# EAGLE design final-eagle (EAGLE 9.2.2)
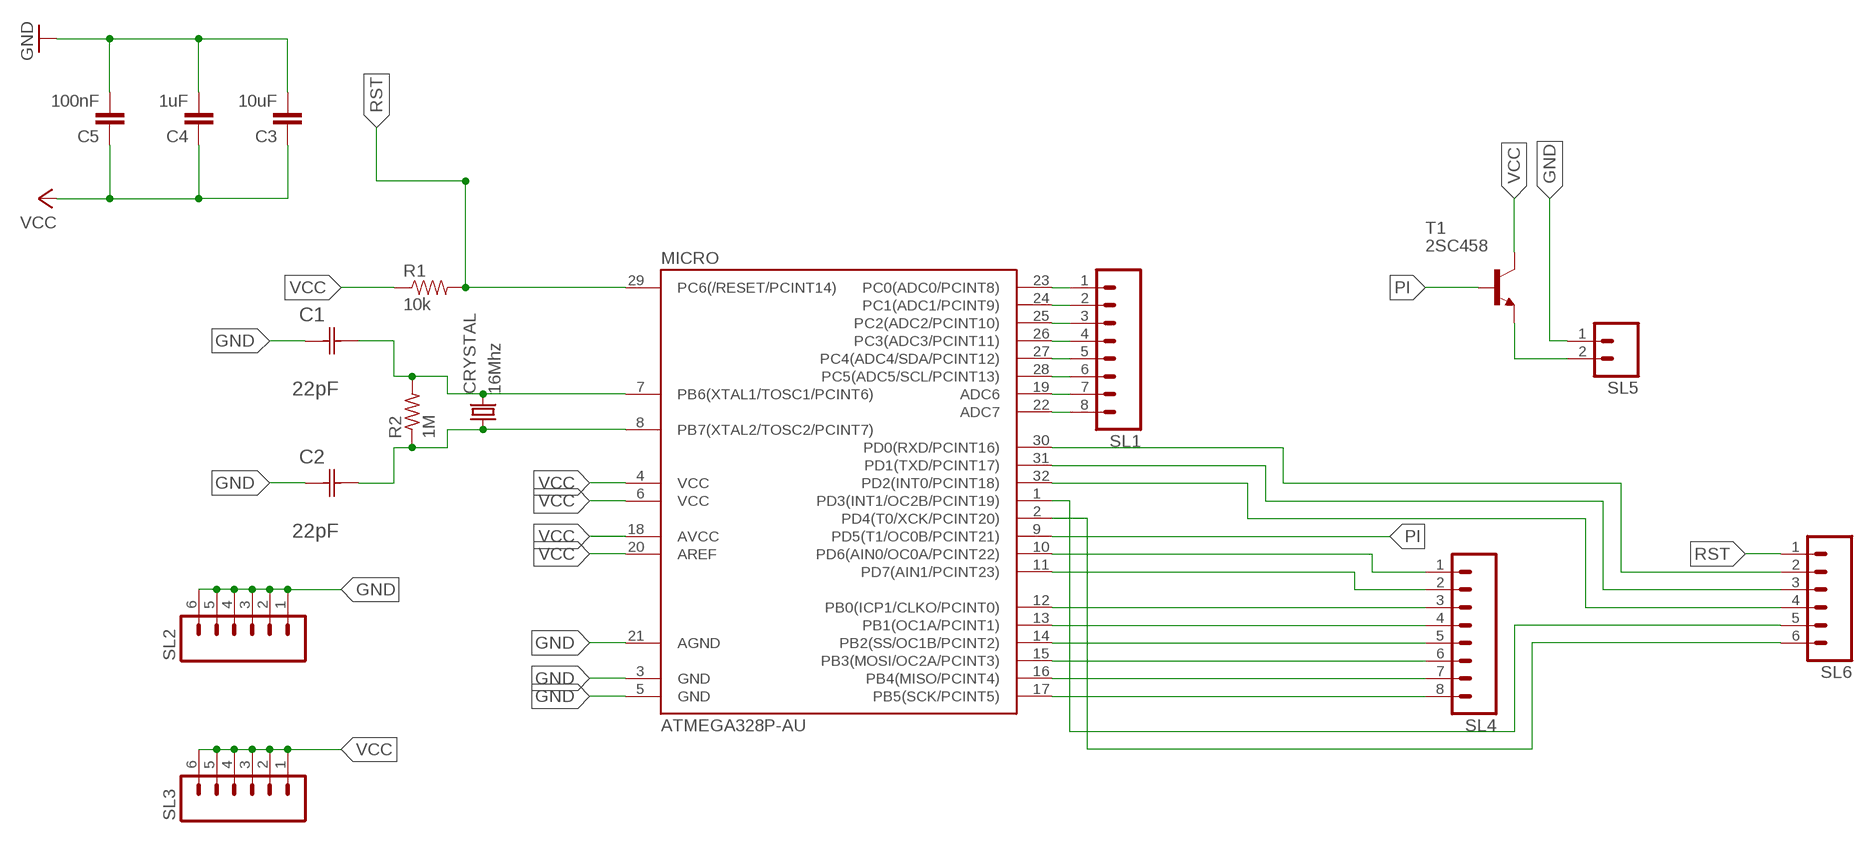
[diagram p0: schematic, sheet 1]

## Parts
C1  22pF  0612ZC225MAT2A  [CAPC3216X178N]
C2  22pF  0612ZC225MAT2A  [CAPC3216X178N]
C3  10uF  CAP1206  [1206]
C4  1uF  CAP1206  [1206]
C5  100nF  CAP1206  [1206]
CRYSTAL  16Mhz  CSM-7X-DU  [CSM-7X-DU]
MICRO  ATMEGA328P-AU  ATMEGA48/88/168-AU  [TQFP32-08]
R1  10k  RESISTOR1206  [1206]
R2  1M  RES-US1206FAB  [R1206FAB]
SL1  M08  [08P]
SL2  M06  [06P]
SL3  M06  [06P]
SL4  M08  [08P]
SL5  M02  [02P]
SL6  M06  [06P]
T1  2SC458  [TO92-ECB]

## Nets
GND: C1.1(C1) C2.1(C1) C3.2 C4.2 C5.2 MICRO.3(GND) MICRO.5(GND) MICRO.21(AGND) SL2.1 SL2.2 SL2.3 SL2.4 SL2.5 SL2.6 SL5.1
N$2: C1.2(C2) CRYSTAL.2 MICRO.7(PB6(XTAL1/TOSC1/PCINT6)) R2.2
N$3: MICRO.23(PC0(ADC0/PCINT8)) SL1.1
N$4: MICRO.10(PD6(AIN0/OC0A/PCINT22)) SL4.1
N$5: MICRO.11(PD7(AIN1/PCINT23)) SL4.2
N$6: MICRO.12(PB0(ICP1/CLKO/PCINT0)) SL4.3
N$7: MICRO.13(PB1(OC1A/PCINT1)) SL4.4
N$8: MICRO.14(PB2(SS/OC1B/PCINT2)) SL4.5
N$9: MICRO.24(PC1(ADC1/PCINT9)) SL1.2
N$10: MICRO.15(PB3(MOSI/OC2A/PCINT3)) SL4.6
N$11: MICRO.16(PB4(MISO/PCINT4)) SL4.7
N$12: MICRO.17(PB5(SCK/PCINT5)) SL4.8
N$13: MICRO.25(PC2(ADC2/PCINT10)) SL1.3
N$14: MICRO.26(PC3(ADC3/PCINT11)) SL1.4
N$15: MICRO.27(PC4(ADC4/SDA/PCINT12)) SL1.5
N$16: MICRO.28(PC5(ADC5/SCL/PCINT13)) SL1.6
N$17: MICRO.19(ADC6) SL1.7
N$18: MICRO.22(ADC7) SL1.8
N$20: MICRO.30(PD0(RXD/PCINT16)) SL6.2
N$21: MICRO.31(PD1(TXD/PCINT17)) SL6.3
N$22: MICRO.32(PD2(INT0/PCINT18)) SL6.4
N$23: MICRO.1(PD3(INT1/OC2B/PCINT19)) SL6.5
N$24: MICRO.2(PD4(T0/XCK/PCINT20)) SL6.6
N$25: SL5.2 T1.E
N$26: C2.2(C2) CRYSTAL.1 MICRO.8(PB7(XTAL2/TOSC2/PCINT7)) R2.1
PI: MICRO.9(PD5(T1/OC0B/PCINT21)) T1.B
RST: MICRO.29(PC6(/RESET/PCINT14)) R1.2 SL6.1
VCC: C3.1 C4.1 C5.1 MICRO.4(VCC) MICRO.6(VCC) MICRO.18(AVCC) MICRO.20(AREF) R1.1 SL3.1 SL3.2 SL3.3 SL3.4 SL3.5 SL3.6 T1.C

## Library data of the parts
C1 C2 = AVX_By_element14_Batch_1:0612ZC225MAT2A: Capacitor 1206; MPN: 0612ZC225MAT2A; OC_FARNELL: -; OC_NEWARK: 12N3209; SUPPLIER: AVX; TOLERANCE: ±20%; VALUE: 2.2µF; VOLTAGERATING: 10V
C3-C5 = 01_SparkFun:CAP: Capacitor
CRYSTAL = 01_FAB_Hello:CSM-7X-DU: SMD CRYSTAL; OC_FARNELL: unknown; OC_NEWARK: unknown
MICRO = atmega8:ATMEGA48/88/168
R1 = 01_SparkFun:RESISTOR: Resistor
R2 = fab:RES-US: Resistor (US Symbol)
SL1 SL4 = con-amp-quick:M08: AMP QUICK CONNECTOR; OC_FARNELL: unknown; OC_NEWARK: unknown
SL2 SL3 SL6 = con-amp-quick:M06: AMP QUICK CONNECTOR; OC_FARNELL: unknown; OC_NEWARK: unknown
SL5 = con-amp-quick:M02: AMP QUICK CONNECTOR; OC_FARNELL: unknown; OC_NEWARK: unknown
T1 = transistor:2SC458: NPN Silicon Epitaxial Planar Transistor Source: SEMTECH ELECTRONICS LTD. ... 2SC458 1.pdf

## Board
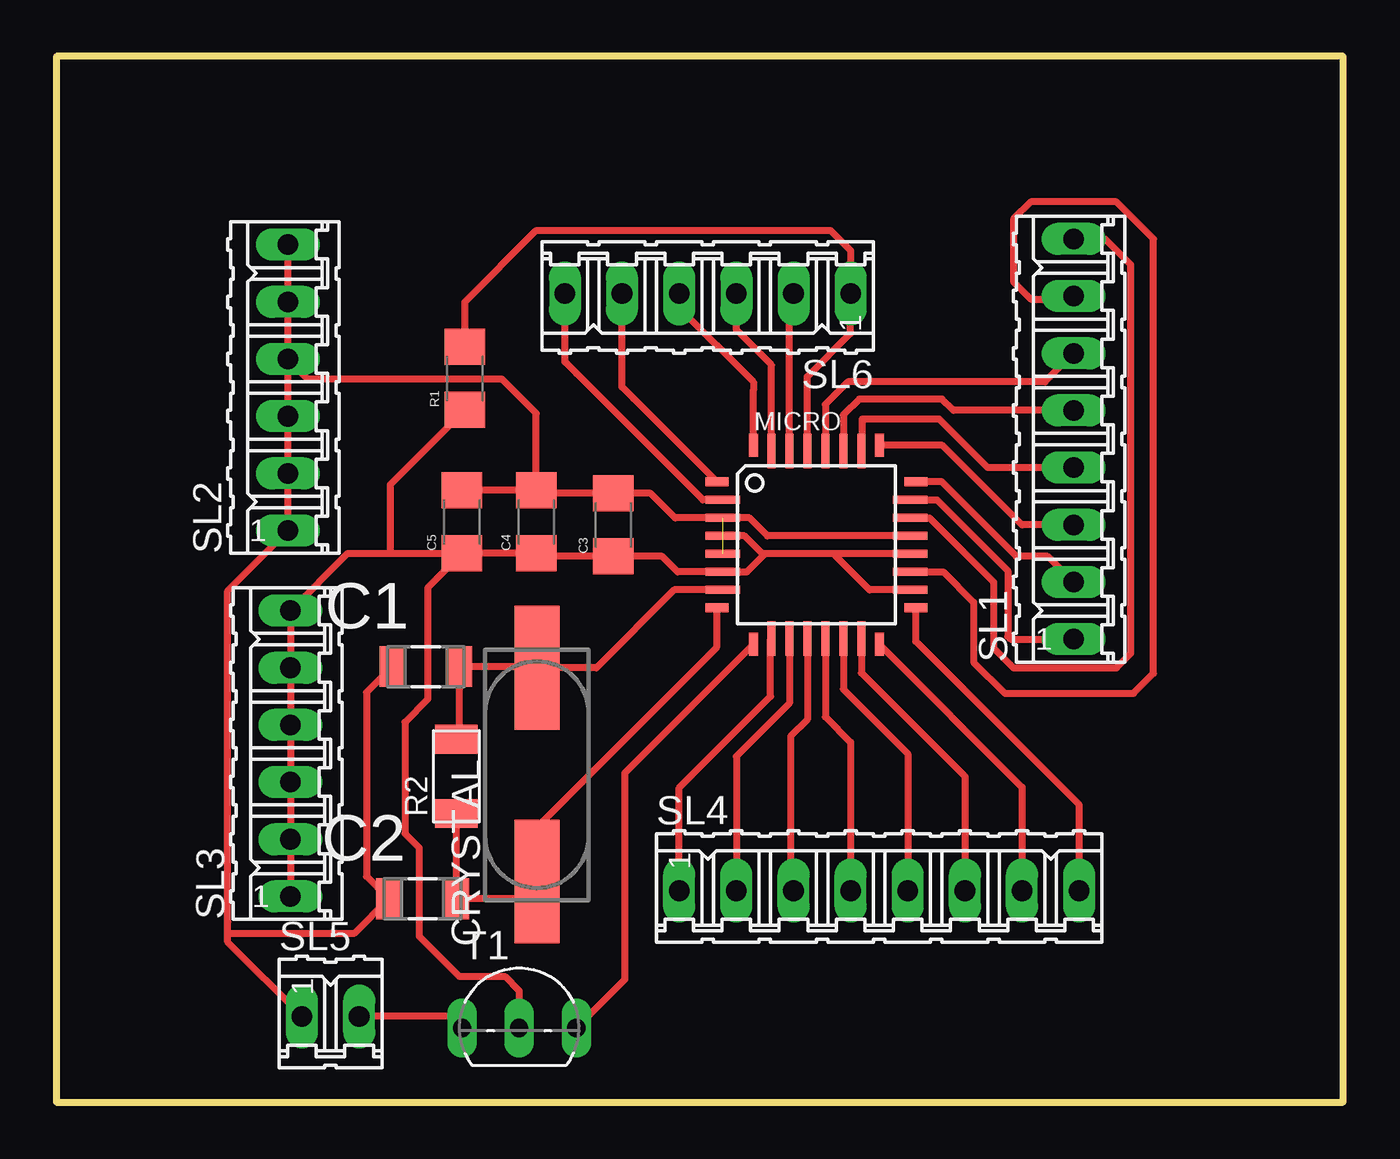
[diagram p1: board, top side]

Size 57.2 x 46.47 mm. Coordinates in mm from the lower left corner, seen from the top.
Outline: 0,0 57.2,0 57.2,46.47 0,46.47 0,0
Copper layers (1*16): Top 0.035mm / dielectric 1.5mm / Bottom 0.035mm
Design rules "default": minimum track width 10mil, minimum drill 24mil, track to track 8mil, track to pad 8mil, pad to pad 8mil, via to via 8mil, smd to smd 8mil, copper to edge 40mil, drill to drill 8mil, minimum pad ring 10mil, minimum via ring 8mil, stop-mask expansion 4mil, vias tented up to drill 0mil, thermal gap 10mil

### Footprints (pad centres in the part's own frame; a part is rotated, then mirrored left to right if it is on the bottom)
CAPC3216X178N = smd 1.118 x 1.803: 1 -1.499,0; 2 1.499,0
1206 = smd 1.6 x 1.8: 1 -1.4,0; 2 1.4,0
CSM-7X-DU = smd 5.5 x 2: 1 -4.75,0; 2 4.75,0
TQFP32-08 = smd 1.016 x 0.406: 1 -4.42,2.8; 8 -4.42,-2.8; 17 4.42,-2.8; 24 4.42,2.8 | smd 1.524 x 0.356: 2 -4.166,2; 3 -4.166,1.2; 4 -4.166,0.4; 5 -4.166,-0.4; 6 -4.166,-1.2; 7 -4.166,-2; 18 4.166,-2; 19 4.166,-1.2; 20 4.166,-0.4; 21 4.166,0.4; 22 4.166,1.2; 23 4.166,2 | smd 0.406 x 1.016: 9 -2.8,-4.42; 16 2.8,-4.42; 25 2.8,4.42; 32 -2.8,4.42 | smd 0.356 x 1.524: 10 -2,-4.166; 11 -1.2,-4.166; 12 -0.4,-4.166; 13 0.4,-4.166; 14 1.2,-4.166; 15 2,-4.166; 26 2,4.166; 27 1.2,4.166; 28 0.4,4.166; 29 -0.4,4.166; 30 -1.2,4.166; 31 -2,4.166
R1206FAB = smd 1.27 x 1.905: 1 -1.651,0; 2 1.651,0
08P = drill 0.914 long: 1 -8.89,0; 2 -6.35,0; 3 -3.81,0; 4 -1.27,0; 5 1.27,0; 6 3.81,0; 7 6.35,0; 8 8.89,0
06P = drill 0.914 long: 1 -6.35,0; 2 -3.81,0; 3 -1.27,0; 4 1.27,0; 5 3.81,0; 6 6.35,0
02P = drill 0.914 long: 1 -1.27,0; 2 1.27,0
TO92-ECB = drill 0.813 long: B 2.54,0; C 0,0; E -2.54,0

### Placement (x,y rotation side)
C1  16.43,19.35 0 top
C2  16.28,9.04 0 top
C3  24.77,25.65 90 top
C4  21.34,25.78 90 top
C5  18.03,25.78 90 top
CRYSTAL  21.36,14.55 90 top
MICRO  33.78,24.77 0 top
R1  18.16,32.16 90 top
R2  17.78,14.48 90 top
SL1  45.21,29.46 90 top
SL2  10.29,31.75 90 top
SL3  10.41,15.49 90 top
SL4  36.58,9.4 0 top
SL5  12.19,3.81 0 top
SL6  28.96,35.94 180 top
T1  20.57,3.3 0 top

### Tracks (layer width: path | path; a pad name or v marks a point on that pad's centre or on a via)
GND  (1 unrouted)
  Top 0.305: MICRO.21 31.6,25.16 30.8,25.96 MICRO.3 27.5,25.96 26.41,27.05 C3.2 21.46,27.05 C4.2 | C4.2 C5.2 | C1.1 13.79,18.21 13.79,10.03 C2.1 13.23,7.49 7.62,7.49 7.62,8 | C4.2 21.34,30.61 19.81,32.13 11.18,32.13 SL2.4 | SL2.6 SL2.5 | 10.29,34.92 SL2.5 | SL2.5 SL2.4 | SL2.4 SL2.3 SL2.2 SL2.1 7.62,22.73 7.62,8 | SL5.1 7.62,7.11 7.62,8
N$2
  Top 0.305: MICRO.7 27.46,22.77 24,19.3 CRYSTAL.2 21.31,19.36 C1.2 17.93,16.28 R2.2
N$3
  Top 0.305: MICRO.23 39.15,26.77 42.29,23.62 42.29,20.7 42.42,20.57 SL1.1
N$4
  Top 0.305: SL4.1 27.69,13.97 31.75,18.03 31.75,20.57 MICRO.10
N$5
  Top 0.305: MICRO.11 32.58,17.72 30.23,15.37 SL4.2
N$6
  Top 0.305: MICRO.12 33.38,17 32.64,16.26 32.64,9.53 SL4.3
N$7
  Top 0.305: MICRO.13 34.18,17.13 35.31,16 SL4.4
N$8
  Top 0.305: MICRO.14 34.98,18.36 37.85,15.49 SL4.5
N$9
  Top 0.305: SL1.2 44.07,24.26 42.67,24.26 39.36,27.57 MICRO.24
N$10
  Top 0.305: MICRO.15 35.78,19.08 40.39,14.48 SL4.6
N$11
  Top 0.305: MICRO.16 42.93,14 SL4.7
N$12
  Top 0.305: SL4.8 45.47,13.21 38.2,20.47 MICRO.17
N$13
  Top 0.305: SL1.3 42.93,25.65 39.4,29.18 MICRO.25
N$14
  Top 0.305: SL1.4 41.4,28.19 39.24,30.35 35.81,30.35 35.81,28.96 MICRO.26
N$15
  Top 0.305: SL1.5 39.88,30.73 39.37,31.24 35.69,31.24 34.98,30.54 MICRO.27
N$16
  Top 0.305: SL1.6 43.94,32 35.18,32 34.18,31.01 MICRO.28
N$17
  Top 0.305: MICRO.19 39.43,23.57 40.77,22.23 40.77,19.56 42.16,18.16 47.88,18.16 48.77,19.05 48.77,38.35 47.12,40.01 43.31,40.01 42.55,39.24 42.55,36.45 43.31,35.69 45.09,35.69 SL1.7
N$18
  Top 0.305: MICRO.22 38.81,25.96 41.66,23.12 41.66,20.19 42.55,19.3 47.12,19.3 47.75,19.94 47.75,37.21 46.61,38.35 SL1.8
N$20
  Top 0.305: MICRO.30 32.58,35.76 SL6.2
N$21
  Top 0.305: MICRO.31 31.78,32.73 31.78,32.77 30.23,34.32 SL6.3
N$22
  Top 0.305: MICRO.32 30.98,31.63 30.98,32 27.69,35.3 SL6.4
N$23
  Top 0.305: MICRO.1 25.65,31.27 25.15,31.78 SL6.5
N$24
  Top 0.305: MICRO.2 28.73,26.77 23.11,32.39 22.61,32.89 SL6.6
N$25
  Top 0.305: 17.91,3.43 T1.E 17.53,3.81 SL5.2
N$26
  Top 0.305: MICRO.8 29.36,20.22 21.36,12.22 CRYSTAL.1 20.6,9.04 C2.2 R2.1
PI
  Top 0.305: T1.B 25.27,5.46 25.27,14.64 MICRO.9
RST
  Top 0.305: MICRO.29 33.38,32.24 35.31,34.16 SL6.1 35.31,37.85 34.42,38.73 21.34,38.73 18.16,35.56 R1.2
VCC
  Top 0.305: MICRO.20 34.54,24.37 | 34.54,24.37 31.5,24.37 | 31.5,24.37 31.39,24.37 30.59,25.16 MICRO.4 | MICRO.18 36.14,22.77 34.54,24.37 | C5.1 C4.1 21.46,24.25 C3.1 26.92,24.26 27.62,23.57 MICRO.6 30.7,23.57 31.5,24.37 | 14.86,24.38 12.95,24.38 SL3.6 SL3.5 SL3.4 SL3.3 SL3.2 SL3.1 10.41,9.02 10.03,8.64 | 14.86,24.38 C5.1 | 14.86,24.38 14.86,27.45 R1.1 | C5.1 16.51,22.86 16.51,17.91 15.49,16.89 15.49,11.94 16.13,11.3 16.13,7.37 17.91,5.59 19.94,5.59 20.57,4.95 T1.C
